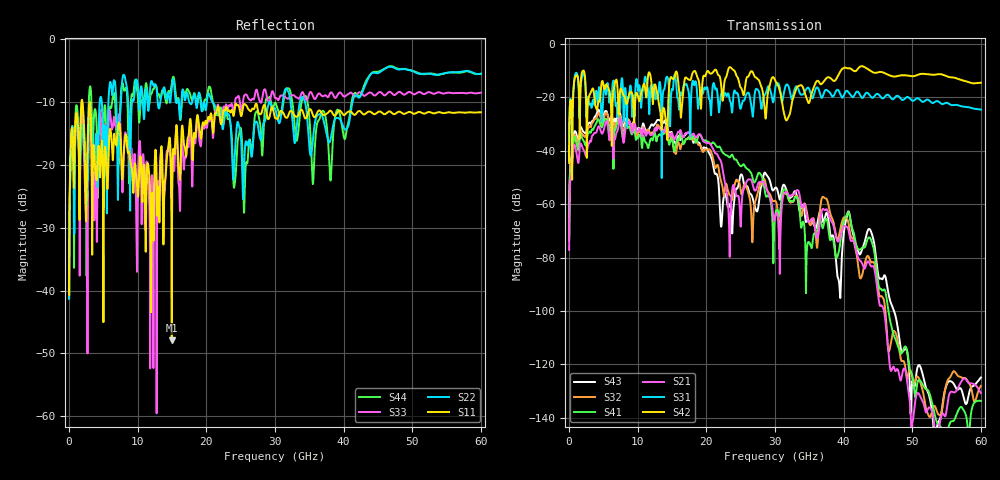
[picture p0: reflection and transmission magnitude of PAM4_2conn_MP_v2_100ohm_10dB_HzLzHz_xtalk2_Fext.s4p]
! Info: Touchstone file created by Circ.  Input file=FAB50GbE_2conn_Midplane_Examax_Topo2_v2_100ohm_10dB_HzLzHz.circ
# Hz S RI R 50
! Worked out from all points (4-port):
!   6000 points, 10 MHz to 60 GHz, reference 50 ohm
!   strongest paths, dB at 10 MHz, 15.01 GHz, 30.01 GHz, 45.01 GHz, 60 GHz:
!     S42: -44.6, -12.9, -13.6, -10.6, -14.5
!     S31: -43.9, -16.8, -17.2, -18.8, -24.6
!     S21: -77.1, -33.4, -64.9, -93.7, -130.7
!     S41: -73.1, -35.2, -64.5, -89.0, -133.7
!     S32: -73.6, -35.5, -58.7, -90.9, -128.1
!     S43: -72.0, -33.6, -53.9, -86.0, -124.9
!   lowest |S11| = -47.9 dB at 14.96 GHz (marker M1), VSWR 1.01, Z = 50.3 - j0.259 ohm
!   |S11| at or under -10 dB: start of sweep to 1.808 GHz; 1.957 GHz to 2.997 GHz (1.04 GHz wide, 42 % of centre); 3.05 GHz to end of sweep
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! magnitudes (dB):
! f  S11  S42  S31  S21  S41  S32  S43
! 10 MHz  -40.7  -44.6  -43.9  -77.1  -73.1  -73.6  -72.0
! 750 MHz  -21.6  -14.1  -13.7  -37.8  -34.9  -34.5  -33.0
! 4.23 GHz  -17.4  -22.2  -20.2  -31.1  -28.2  -26.1  -24.7
! 14.96 GHz  -47.9  -12.6  -16.9  -33.3  -35.3  -34.9  -33.1
! 23.36 GHz  -11.3  -8.8  -20.5  -73.2  -42.5  -56.5  -60.5
! 34.7 GHz  -12.1  -21.1  -16.5  -65.5  -75.6  -63.8  -66.0
! 60 GHz  -11.6  -14.5  -24.6  -130.7  -133.7  -128.1  -124.9
